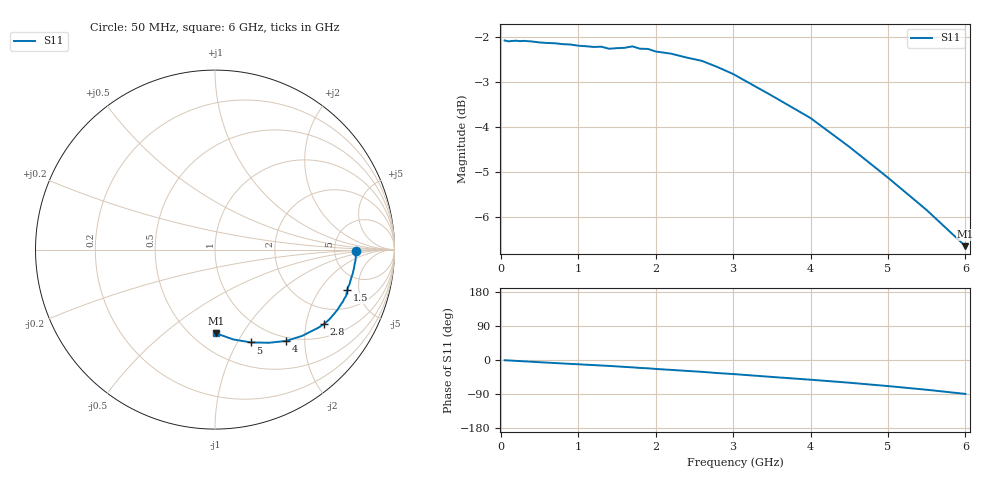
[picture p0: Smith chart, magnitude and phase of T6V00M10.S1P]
! SIEMENS Discrete & RF Semiconductors
! BAT62
! Si Schottky Diode in SOT143
! IF = 0.1 mA
! S-Parameters:  February  1997
# GHz  S  MA  R  50
!  f  S11
! GHz  MAG  ANG
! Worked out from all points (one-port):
!   34 points, 50 MHz to 6 GHz, reference 50 ohm
!   lowest |S11| = -6.6 dB at 6 GHz (marker M1), VSWR 2.74, Z = 32.4 - j38.5 ohm
!   |S11| at or under -10 dB: nowhere
!   S11 on the Smith chart (normalised r, x): 50 MHz: 8.35, -0.36; 1.5 GHz: 3.41, -3.77; 2.8 GHz: 1.40, -2.53; 4 GHz: 0.94, -1.64; 5 GHz: 0.76, -1.14; 6 GHz: 0.65, -0.77
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0.05  0.7865 -0.6
0.1  0.7847 -1.2
0.15  0.7855 -1.7
0.2  0.7859 -2.4
0.4  0.7845 -4.6
0.5  0.7825 -5.8
0.8  0.7792 -9.1
0.9  0.7784 -10.3
1  0.7761 -11.2
1.3  0.7741 -14.6
1.4  0.77 -15.6
1.5  0.7713 -16.9
1.6  0.7719 -18.2
1.7  0.7748 -19.4
1.8  0.7701 -20.9
1.9  0.7698 -21.9
2  0.7647 -23.6
2.2  0.7605 -26.1
2.4  0.753 -28.7
2.6  0.7466 -31.3
2.8  0.735 -34.5
3  0.7221 -37.0
3.5  0.6834 -44.7
4  0.6456 -52.0
4.5  0.6001 -59.9
5  0.5547 -68.8
5.5  0.5108 -78.5
6  0.4659 -89.5
